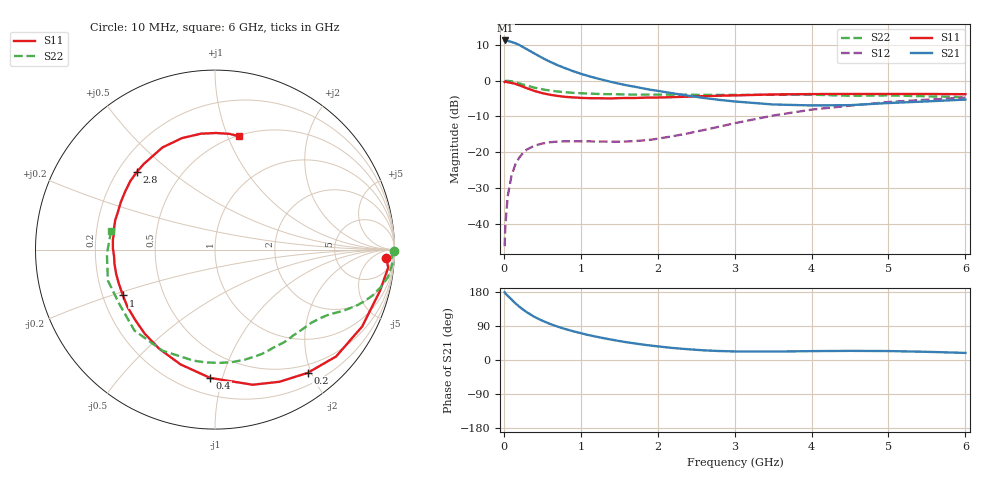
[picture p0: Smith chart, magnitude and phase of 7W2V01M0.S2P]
! Infineon Technologies  Discrete & RF Semiconductors
! BFS17W
! Si NPN RF Bipolar Junction Transistor in SOT323
! VCE = 2 V  IC = 1 mA
! Common Emitter S-Parameters:  August  1999
# GHz  S  MA  R  50
!  f  S11  S21  S12  S22
! GHz  MAG  ANG  MAG  ANG  MAG  ANG  MAG  ANG
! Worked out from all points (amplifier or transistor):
!   36 points, 10 MHz to 6 GHz, reference 50 ohm
!   highest |S21| = 11.2 dB at 20 MHz (marker M1)
!   |S21| within 3 dB of that: start of sweep to 345.1 MHz
!   unconditionally stable (mu >= 1): 999.1 MHz to end of sweep
!   at 250 MHz: K = 0.27, MSG = 14.8 dB, |S12| = -20.2 dB
!   at 1.4 GHz: K = 1.31, MAG = 5.0 dB, |S12| = -17.1 dB
!   at 6 GHz: K = 1.11, MAG = -2.3 dB, |S12| = -4.8 dB
!   S11 on the Smith chart (normalised r, x): 10 MHz: 21, -22; 200 MHz: 0.37, -1.95; 400 MHz: 0.31, -0.91; 1 GHz: 0.29, -0.22; 2.8 GHz: 0.28, +0.38; 6 GHz: 0.51, +1.10
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0.01  0.9558 -2.7  3.588 178.7  0.0049 88.4  0.9999 -0.4
0.02  0.9701 -6.0  3.625 175.9  0.0096 90.3  0.9856 -1.8
0.05  0.9472 -14.1  3.565 169.4  0.0242 81.9  0.9912 -4.7
0.1  0.925 -27.6  3.458 159.7  0.0475 73.7  0.9756 -9.1
0.15  0.9 -41.4  3.314 149.7  0.0676 66.3  0.9447 -13.0
0.2  0.8591 -53.1  3.142 141.0  0.0843 60.5  0.9127 -16.4
0.25  0.8193 -64.0  2.928 133.1  0.0979 54.0  0.8788 -19.2
0.3  0.7817 -74.4  2.734 125.9  0.1093 49.7  0.8492 -21.5
0.4  0.7156 -92.1  2.376 113.5  0.1239 41.8  0.7947 -25.3
0.5  0.6679 -106.7  2.073 103.7  0.1324 36.7  0.7549 -27.9
0.6  0.6339 -119.4  1.83 95.2  0.1381 33.2  0.7254 -30.2
0.8  0.5924 -138.8  1.484 81.6  0.1422 29.0  0.6874 -35.0
1  0.5731 -153.5  1.245 70.9  0.1421 27.9  0.6665 -39.6
1.1  0.5683 -160.5  1.156 65.8  0.1422 28.2  0.6586 -42.4
1.6  0.5715 174.5  0.857 46.7  0.1413 35.5  0.6386 -56.5
2.2  0.5876 153.3  0.663 31.6  0.1676 50.1  0.6355 -75.1
2.8  0.614 135.2  0.538 23.7  0.2275 57.7  0.6305 -94.8
3.5  0.6401 117.2  0.464 22.2  0.3251 56.3  0.6347 -117.5
4  0.6479 106.5  0.45 23.4  0.3931 50.8  0.6361 -134.9
4.5  0.6506 96.9  0.454 24.1  0.4466 44.5  0.6133 -150.6
5.5  0.65 82.9  0.512 21.6  0.5411 32.1  0.6027 -177.8
6  0.6454 77.9  0.543 18.7  0.5773 26.3  0.5882 170.1
